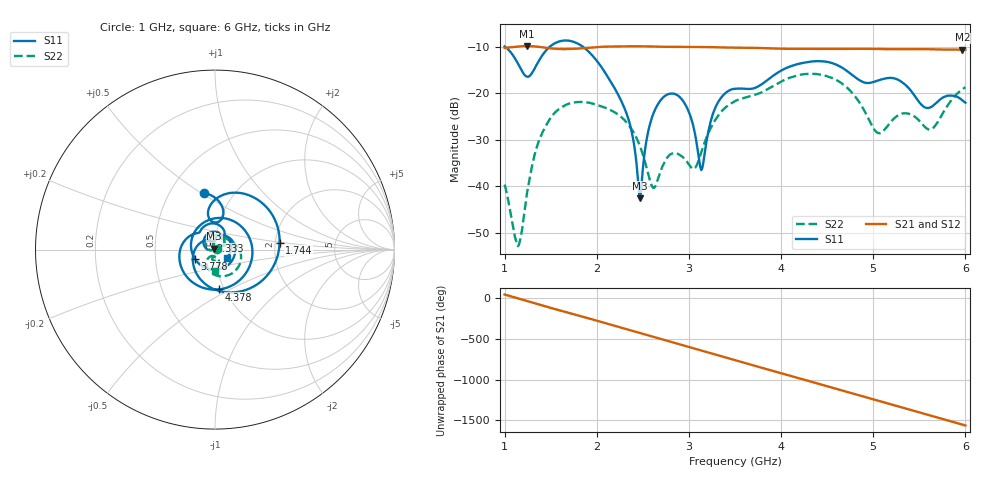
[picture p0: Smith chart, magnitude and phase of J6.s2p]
!Agilent Technologies,E8364B,MY43040528,A.07.50.67
!Agilent E8364B: A.07.50.67
!Date: Sunday, March 01, 2026 15:26:25
!Correction: S11(Full 2 Port(1,2))
!S21(Full 2 Port(1,2))
!S12(Full 2 Port(1,2))
!S22(Full 2 Port(1,2))
!S2P File: Measurements: S11, S21, S12, S22:
# Hz S  dB  R 50
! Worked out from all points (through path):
!   451 points, 1 GHz to 6 GHz, reference 50 ohm
!   highest |S21| = -9.76 dB at 1.244 GHz (marker M1); lowest = -10.6 dB at 5.967 GHz (marker M2)
!   group delay of S21, straight-line fit = 893 ps
!   lowest |S11| = -42.6 dB at 2.467 GHz (marker M3), VSWR 1.01, Z = 49.5 + j0.527 ohm
!   |S11| at or under -10 dB: 1.011 GHz to 1.485 GHz (474.5 MHz wide, 38 % of centre); 1.856 GHz to end of sweep
!   |S22| runs from -53.0 to -15.8 dB; largest |S21 - S12| = 0.0015
!   S11 on the Smith chart (normalised r, x): 1 GHz: 0.73, +0.51; 1.744 GHz: 2.11, +0.18; 2.333 GHz: 0.94, +0.10; 3.778 GHz: 0.79, -0.08; 4.378 GHz: 0.94, -0.44; 6 GHz: 1.14, -0.10
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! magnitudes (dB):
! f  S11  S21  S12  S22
! 1 GHz  -9.8  -10.1  -10.2  -39.7
! 1.144 GHz  -13.5  -9.9  -9.9  -53.0
! 1.244 GHz  -16.4  -9.8  -9.8  -41.3
! 1.433 GHz  -11.1  -10.1  -10.1  -27.5
! 1.744 GHz  -8.8  -10.4  -10.4  -22.0
! 1.844 GHz  -9.8  -10.2  -10.3  -21.8
! 2.333 GHz  -24.9  -9.8  -9.8  -26.5
! 2.467 GHz  -42.6  -9.8  -9.8  -31.3
! 2.6 GHz  -25.1  -9.9  -9.9  -40.0
! 2.667 GHz  -22.2  -9.9  -9.9  -38.3
! 2.933 GHz  -21.5  -9.9  -10.0  -33.7
! 3.133 GHz  -36.5  -10.0  -10.0  -32.8
! 3.289 GHz  -23.0  -10.0  -10.1  -25.6
! 3.5 GHz  -19.0  -10.1  -10.1  -21.7
! 3.778 GHz  -18.2  -10.2  -10.2  -19.9
! 4.344 GHz  -13.1  -10.4  -10.4  -15.8
! 4.378 GHz  -13.0  -10.4  -10.4  -15.8
! 5.044 GHz  -17.2  -10.4  -10.4  -28.5
! 5.167 GHz  -16.6  -10.4  -10.5  -26.7
! 5.633 GHz  -22.9  -10.5  -10.5  -27.7
! 5.967 GHz  -21.5  -10.6  -10.6  -19.1
! 6 GHz  -22.0  -10.6  -10.6  -18.6
